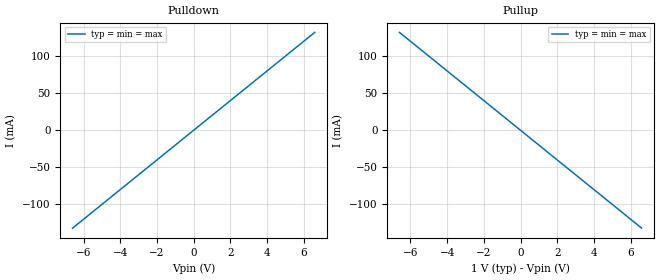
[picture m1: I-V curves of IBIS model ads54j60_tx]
[IBIS Ver]   5.0
[File Name]   ads54j60_tx.ibs
[File Rev]   1.0
[Component]   ads54j60_tx
[Manufacturer] My Company
[Package]
R_pkg  0.0   NA   NA
L_pkg  0.0   NA   NA
C_pkg  0.0   NA   NA
[Pin]   signal_name   model_name   R_pin L_pin  C_pin
1p   ads54j60_tx_p   ads54j60_tx
1n   ads54j60_tx_n   ads54j60_tx
[Diff_Pin] inv_pin vdiff tdelay_typ tdelay_min tdelay_max
1p   1n   NA   NA   NA   NA
| Models and submodels in the file (1): ads54j60_tx (Output)
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[Model] ads54j60_tx
Model_type Output
C_comp 0p 0p 0p
Cref = 0
Vref = 0.5
Rref = 50
Vmeas = 0.5
[Temperature_Range] 25 125 0
[Voltage Range] 1.0 1.0 1.0
[Algorithmic Model]
Executable Windows_cl16.00.40219.01_64 ads54j60_tx_x64.dll ads54j60_tx.ami
Executable Windows_cl16.00.40219.01_32 ads54j60_tx.dll ads54j60_tx.ami
Executable Linux_gcc4.7.2_64 ads54j60_tx_x64.so ads54j60_tx.ami
[End Algorithmic Model]
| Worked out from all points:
|   slope of the pulldown table from 0 to 0.15 V, typ, clamps not added: 50 ohm
|   slope of the pullup table from 0 to 0.15 V, typ, clamps not added: 50 ohm
[Pulldown]
-6.6V     -132mA     -132mA     -132mA
0V        0A         0A         0A
6.6V      132mA      132mA      132mA
[Pullup]
-6.6V     132mA      132mA      132mA
0V        0A         0A         0A
6.6V      -132mA     -132mA     -132mA
[GND Clamp]
-6.6V     0A         0A         0A
0V        0A         0A         0A
6.6V      0A         0A         0A
[Power Clamp]
-6.6V     0A         0A         0A
0V        0A         0A         0A
6.6V      0A         0A         0A
[Ramp]
dV/dt_r 0.3/1.5p 0.3/1.5p 0.3/1.5p
dV/dt_f 0.3/1.5p 0.3/1.5p 0.3/1.5p
